|Texas Instruments Incorporated
|tmux1308, 1 Data Lane 8_1x1 5V Precision mux
[IBIS Ver]   4.1
[File name]   tmux1308.ibs
[Date]   07/12/22
[File Rev]   1.0
[Source]
| Texas Instruments Incorporated.
| ASC-INT-MPD
| 12500 TI Blvd
| Dallas, TX - 75243
[Notes]   Revision History:
| Rev 1.0: 07/12/22
| - Initial version of the model
| - Model generated from simulations in SPECTRE
| - C_comp although listed in numerical order of value are
|   obtained from varying PVT conditions. For PVT conditions for
|   each specific value refer the buffer description under
|   respective [Model]. IBIS model user is responsible for using
|   appropriate C_comp to simulate for Signal Integrity.
[Disclaimer]
| This model is designed as an aid for customers of Texas Instruments.
| TI and its licensors and suppliers make no warranties, either expressed
| or implied, with respect to this  model, including the warranties of
| merchantability or fitness for a particular purpose. The model is
| provided solely on an "as is" basis. The entire risk as to its quality
| and performance is with the customer.
| This model is subject to change without notice. Texas Instruments
| Incorporated is not responsible for updating this model.
[Copyright]
(C) Copyright 2022 Texas Instruments Incorporated.All rights reserved.
|  Component TMUX1308PW 16-pin - PW package
|  Part # TMUX1308PW
[Component]   TMUX1308PW
[Manufacturer]  TI
[Package]
|   typ   min   max
R_pkg   0.0668   NA   NA
L_pkg   2.1992nH   NA   NA
C_pkg   0.2884pF   NA   NA
[Pin]   signal_name   model_name
   1   S4   sterm
   2   S6   sterm
   3   D   dterm
   4   S7   sterm
   5   S5   sterm
   6   ENZ_5P5_PAD   inbuf
   7   NC   nc
   8   GND   gnd
   9   A2   inbuf
   10   A1   inbuf
   11   A0   inbuf
   12   S3   sterm
   13   S0   sterm
   14   S1   sterm
   15   S2   sterm
   16   VDD   power
[Series Switch Groups]
On 1 /
On 2 /
On 3 /
On 4 /
On 5 /
On 6 /
On 7 /
On 8 /
Off 1 /
[Series Pin Mapping]  pin_2 model_name function_table_group
  13   3   switch_1.8   1
  14   3   switch_1.8   2
  15   3   switch_1.8   3
  12   3   switch_1.8   4
   1   3   switch_1.8   5
   5   3   switch_1.8   6
   2   3   switch_1.8   7
   4   3   switch_1.8   8
|  13   3   switch_3.3   1
|  14   3   switch_3.3   2
|  15   3   switch_3.3   3
|  12   3   switch_3.3   4
|   1   3   switch_3.3   5
|   5   3   switch_3.3   6
|   2   3   switch_3.3   7
|   4   3   switch_3.3   8
|  13   3   switch_2.5   1
|  14   3   switch_2.5   2
|  15   3   switch_2.5   3
|  12   3   switch_2.5   4
|   1   3   switch_2.5   5
|   5   3   switch_2.5   6
|   2   3   switch_2.5   7
|   4   3   switch_2.5   8
|  13   3   switch_5   1
|  14   3   switch_5   2
|  15   3   switch_5   3
|  12   3   switch_5   4
|   1   3   switch_5   5
|   5   3   switch_5   6
|   2   3   switch_5   7
|   4   3   switch_5   8
|  Component TMUX1308DYY 16-pin - DYY package
|  Part # TMUX1308DYY
[Component]   TMUX1308DYY
[Manufacturer]  TI
[Package]
|   typ   min   max
R_pkg   0.0668   NA   NA
L_pkg   2.1992nH   NA   NA
C_pkg   0.2884pF   NA   NA
[Pin]   signal_name   model_name
   1   S4   sterm
   2   S6   sterm
   3   D   dterm
   4   S7   sterm
   5   S5   sterm
   6   ENZ_5P5_PAD inbuf
   7   NC   nc
   8   GND   gnd
   9   A2   inbuf
   10   A1   inbuf
   11   A0   inbuf
   12   S3   sterm
   13   S0   sterm
   14   S1   sterm
   15   S2   sterm
   16   VDD   power
[Series Switch Groups]
On 1 /
On 2 /
On 3 /
On 4 /
On 5 /
On 6 /
On 7 /
On 8 /
Off 1 /
[Series Pin Mapping]  pin_2 model_name function_table_group
  13   3   switch_1.8   1
  14   3   switch_1.8   2
  15   3   switch_1.8   3
  12   3   switch_1.8   4
   1   3   switch_1.8   5
   5   3   switch_1.8   6
   2   3   switch_1.8   7
   4   3   switch_1.8   8
|  13   3   switch_3.3   1
|  14   3   switch_3.3   2
|  15   3   switch_3.3   3
|  12   3   switch_3.3   4
|   1   3   switch_3.3   5
|   5   3   switch_3.3   6
|   2   3   switch_3.3   7
|   4   3   switch_3.3   8
|  13   3   switch_2.5   1
|  14   3   switch_2.5   2
|  15   3   switch_2.5   3
|  12   3   switch_2.5   4
|   1   3   switch_2.5   5
|   5   3   switch_2.5   6
|   2   3   switch_2.5   7
|   4   3   switch_2.5   8
|  13   3   switch_5   1
|  14   3   switch_5   2
|  15   3   switch_5   3
|  12   3   switch_5   4
|   1   3   switch_5   5
|   5   3   switch_5   6
|   2   3   switch_5   7
|   4   3   switch_5   8
|  Component TMUX1308BQB 16-pin - BQB package
|  Part # TMUX1308BQB
[Component]   TMUX1308BQB
[Manufacturer]  TI
[Package]
|   typ   min   max
R_pkg   0.0668   NA   NA
L_pkg   2.1992nH   NA   NA
C_pkg   0.2884pF   NA   NA
[Pin]   signal_name   model_name
   1   S4   sterm
   2   S6   sterm
   3   D   dterm
   4   S7   sterm
   5   S5   sterm
   6   ENZ_5P5_PAD   inbuf
   7   NC   nc
   8   GND   gnd
   9   A2   inbuf
   10   A1   inbuf
   11   A0   inbuf
   12   S3   sterm
   13   S0   sterm
   14   S1   sterm
   15   S2   sterm
   16   VDD   power
[Series Switch Groups]
On 1 /
On 2 /
On 3 /
On 4 /
On 5 /
On 6 /
On 7 /
On 8 /
Off 1 /
[Series Pin Mapping]  pin_2 model_name function_table_group
  13   3   switch_1.8   1
  14   3   switch_1.8   2
  15   3   switch_1.8   3
  12   3   switch_1.8   4
   1   3   switch_1.8   5
   5   3   switch_1.8   6
   2   3   switch_1.8   7
   4   3   switch_1.8   8
|  13   3   switch_3.3   1
|  14   3   switch_3.3   2
|  15   3   switch_3.3   3
|  12   3   switch_3.3   4
|   1   3   switch_3.3   5
|   5   3   switch_3.3   6
|   2   3   switch_3.3   7
|   4   3   switch_3.3   8
|  13   3   switch_2.5   1
|  14   3   switch_2.5   2
|  15   3   switch_2.5   3
|  12   3   switch_2.5   4
|   1   3   switch_2.5   5
|   5   3   switch_2.5   6
|   2   3   switch_2.5   7
|   4   3   switch_2.5   8
|  13   3   switch_5   1
|  14   3   switch_5   2
|  15   3   switch_5   3
|  12   3   switch_5   4
|   1   3   switch_5   5
|   5   3   switch_5   6
|   2   3   switch_5   7
|   4   3   switch_5   8
[Model Selector] dterm
dterm_1.8 Use for operation at 1V
dterm_3.3 Use for operation at 3V
dterm_2.5 Use for operation at 2V
dterm_5 Use for operation at 5V
[Model Selector] sterm
sterm_1.8 Use for operation at 1V
sterm_3.3 Use for operation at 3V
sterm_2.5 Use for operation at 2V
sterm_5 Use for operation at 5V
[Model Selector] inbuf
inbuf_1.8 Use for operation at 1V
inbuf_3.3 Use for operation at 3V
inbuf_2.5 Use for operation at 2V
inbuf_5 Use for operation at 5V
| switch_1.8
[Model]   switch_1.8
Model_type   Series_switch
|   typ   min   max
C_comp   6.362683e-13   NA   NA
[Voltage Range]   1.8   NA   NA
[Power Clamp Reference]   1.8   NA   NA
[Temperature Range]   27   NA   NA
[On]
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[Off]
|   typ   min   max
[R Series]   10G   NA   NA
| switch_3.3
[Model]   switch_3.3
Model_type   Series_switch
|   typ   min   max
C_comp   1.008417e-12   NA   NA
[Voltage Range]   3.3   NA   NA
[Power Clamp Reference]   3.3   NA   NA
[Temperature Range]   27   NA   NA
[On]
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[Off]
|   typ   min   max
[R Series]   10G   NA   NA
| switch_2.5
[Model]   switch_2.5
Model_type   Series_switch
|   typ   min   max
C_comp   1.008417e-12   NA   NA
[Voltage Range]   2.5   NA   NA
[Power Clamp Reference]   2.5   NA   NA
[Temperature Range]   27   NA   NA
[On]
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[Off]
|   typ   min   max
[R Series]   10G   NA   NA
| switch_5
[Model]   switch_5
Model_type   Series_switch
|   typ   min   max
C_comp   1.008417e-12   NA   NA
[Voltage Range]   5   NA   NA
[Power Clamp Reference]   5   NA   NA
[Temperature Range]   27   NA   NA
[On]
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[Off]
|   typ   min   max
[R Series]   10G   NA   NA
| Models and submodels in the file (16): dterm_1.8 (Terminator), dterm_3.3 (Terminator), dterm_2.5 (Terminator), dterm_5 (Terminator), switch_1.8 (Series_switch), switch_3.3 (Series_switch), switch_2.5 (Series_switch), switch_5 (Series_switch), sterm_1.8 (Terminator), sterm_3.3 (Terminator), sterm_2.5 (Terminator), sterm_5 (Terminator), inbuf_1.8 (Input), inbuf_3.3 (Input), inbuf_2.5 (Input), inbuf_5 (Input)
